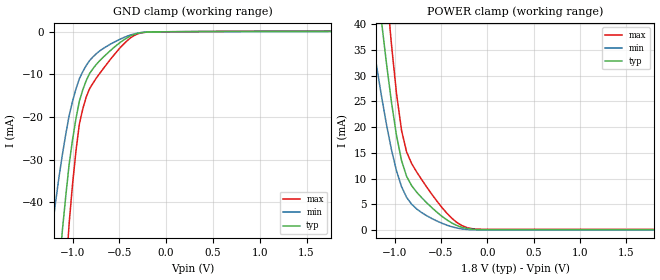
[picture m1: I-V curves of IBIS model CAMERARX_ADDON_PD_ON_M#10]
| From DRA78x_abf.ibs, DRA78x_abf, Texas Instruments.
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| Model based on original model for CAMERARX_ADDON
|   Sub model CAMERARX_ADDON_PD_ON
[model]   CAMERARX_ADDON_PD_ON_M#10
|[Description]  [1.8V-INPUT-X-X]
|   , ,
|[Input Load]
|[Output Drive]
|Voltage   1.8V
|Mode   INPUT
Model_type   Input
Polarity   Non-Inverting
Vinl =  0.63
Vinh =  1.17
C_comp   1.75p   1.5p   2p
[Model Spec]
Vinl   0.63   0.567   0.6615
Vinh   1.17   1.053   1.2285
[Temperature Range]   25   125   -40
[Voltage Range]   1.8   1.62   1.92
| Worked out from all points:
|   GND clamp passes 1 mA (typ) near -0.38 V on its own axis
|   POWER clamp passes 1 mA (typ) near -0.34 V on its own axis
[POWER_clamp]
-1.8V     156.8mA    109.4mA    217.7mA
-1.255V   58.61mA    38.51mA    83.64mA
-1.145V   40.74mA    26.16mA    58.74mA
-1.127V   37.98mA    24.3mA     54.83mA
-1.055V   27.39mA    17.28mA    39.71mA
-981.8mV  18.38mA    11.52mA    26.53mA
-927.3mV  13.51mA    8.445mA    19.36mA
-872.7mV  10.45mA    6.379mA    15.19mA
-654.5mV  5.319mA    2.808mA    8.366mA
-381.8mV  1.388mA    664uA      2.294mA
-163.6mV  213.4uA    86.79uA    305.9uA
1.8V      110.1uA    53.6uA     169.3uA
[GND_clamp]
-1.8V     -252.1mA   -161mA     -379.9mA
-1.218V   -75mA      -46.17mA   -113.7mA
-1.109V   -46.69mA   -28.88mA   -69.6mA
-1.036V   -31.09mA   -19.65mA   -44.93mA
-963.6mV  -20.36mA   -13.4mA    -27.98mA
-927.3mV  -16.27mA   -11.01mA   -21.64mA
-854.5mV  -11.47mA   -7.933mA   -15.33mA
-818.2mV  -9.793mA   -6.756mA   -13.36mA
-636.4mV  -5.221mA   -3.433mA   -7.63mA
-418.2mV  -1.433mA   -1.049mA   -2.128mA
-272.7mV  -219.5uA   -198.1uA   -266.5uA
1.764V    108.8uA    78.64uA    165.8uA
